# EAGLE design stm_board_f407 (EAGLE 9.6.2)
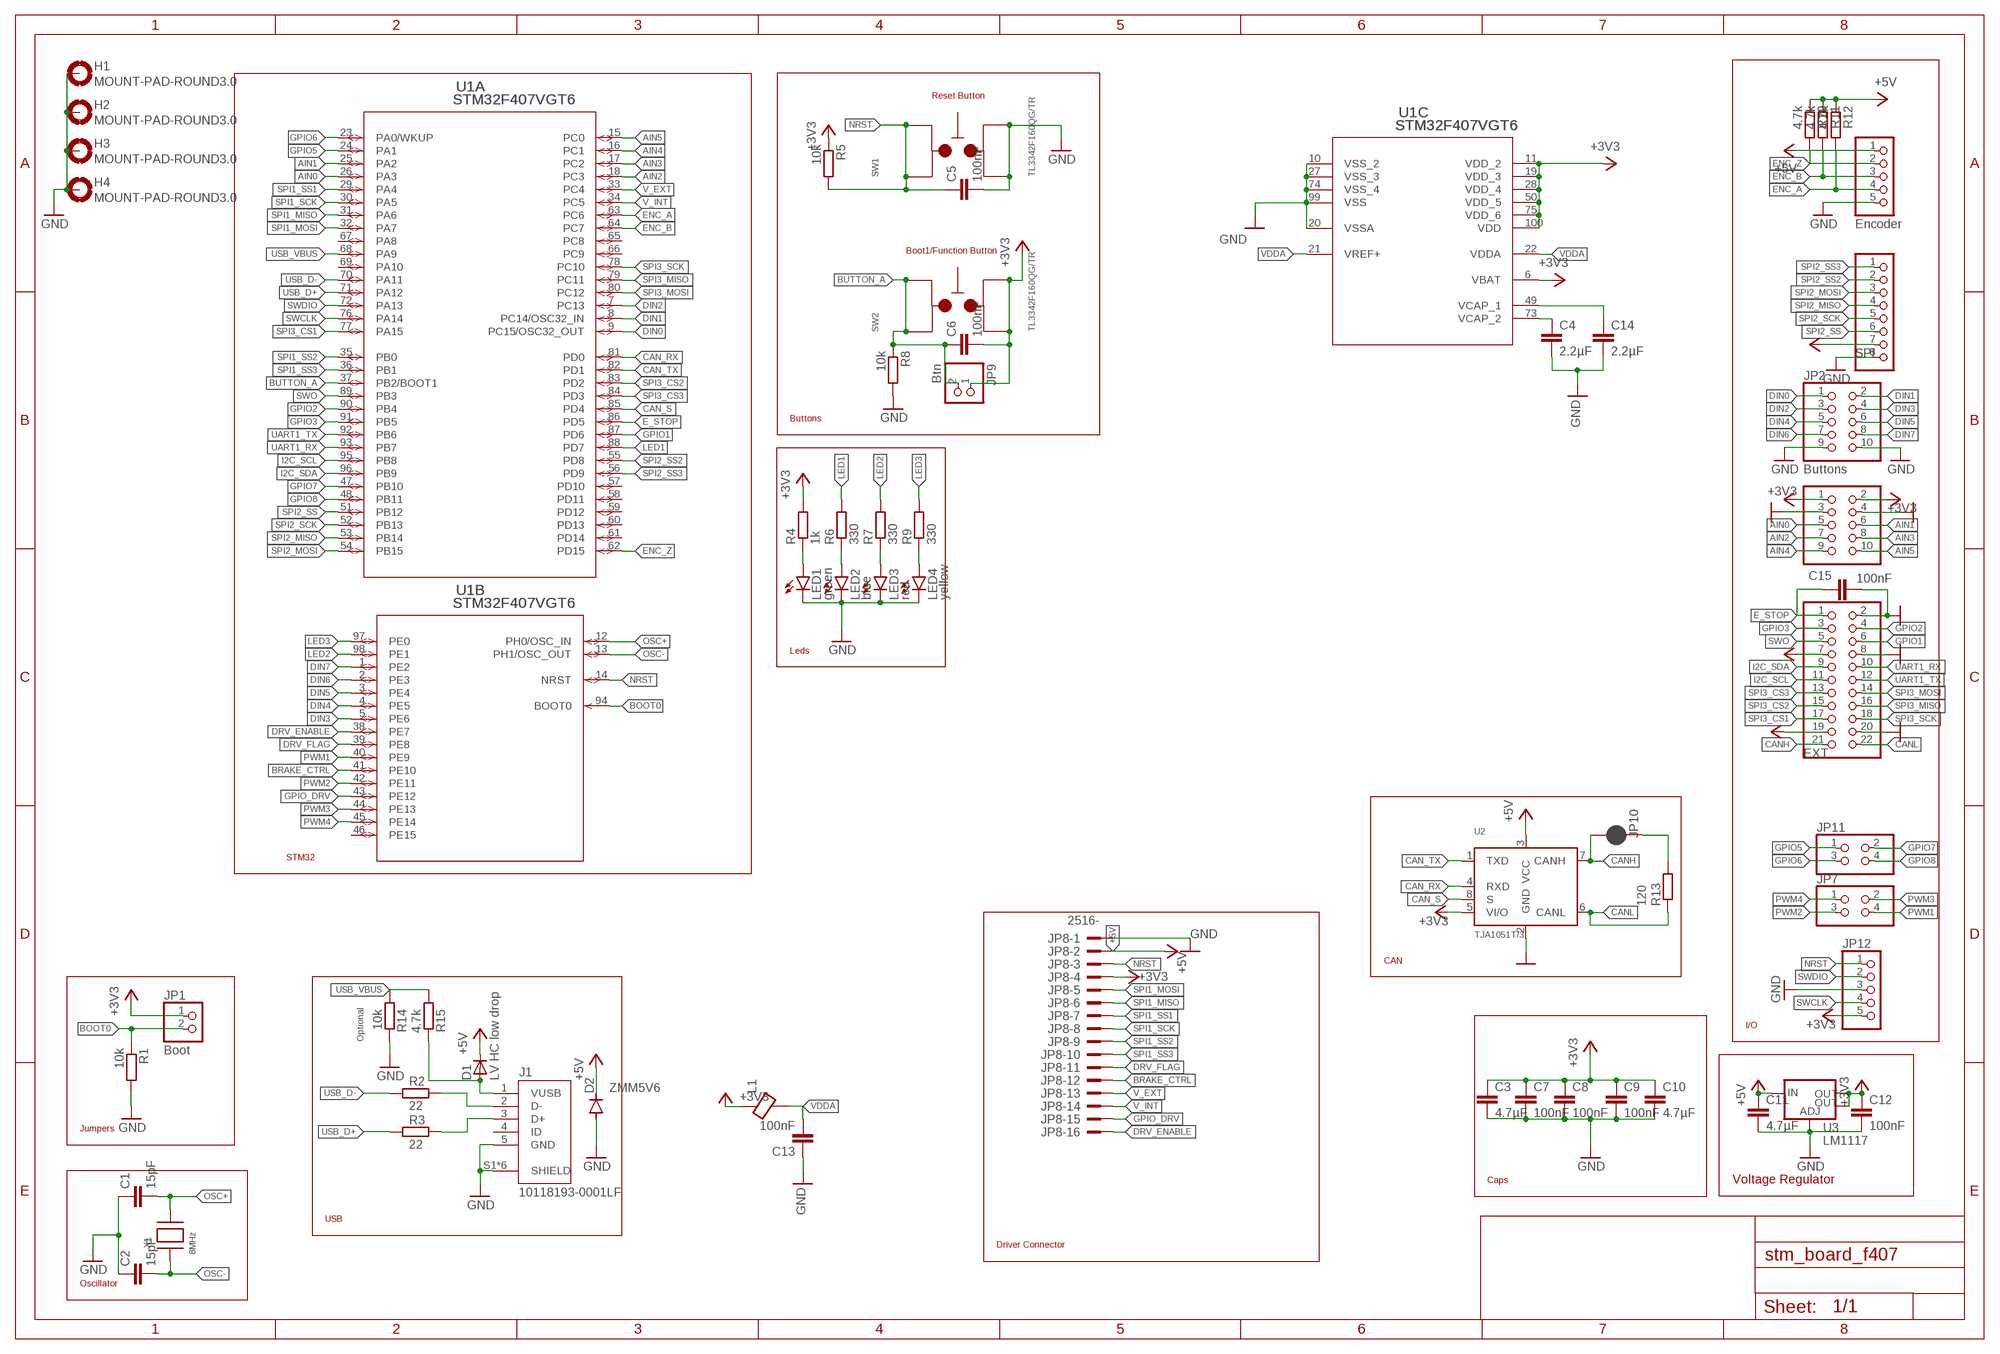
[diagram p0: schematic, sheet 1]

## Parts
C1  15pF  C-EUC0603  [C0603]
C2  15pF  C-EUC0603  [C0603]
C3  4.7µF  C-EUC0805  [C0805]
C4  2.2µF  C-EUC0603  [C0603]
C5  100nF  C-EUC0603  [C0603]
C6  100nF  C-EUC0603  [C0603]
C7  100nF  C-EUC0603  [C0603]
C8  100nF  C-EUC0603  [C0603]
C9  100nF  C-EUC0603  [C0603]
C10  4.7µF  C-EUC0805  [C0805]
C11  4.7µF  C-EUC0805  [C0805]
C12  100nF  C-EUC0603  [C0603]
C13  100nF  C-EUC0603  [C0603]
C14  2.2µF  C-EUC0603  [C0603]
C15  100nF  C-EUC0603  [C0603]
D1  LV HC low drop  DIODESMA  [SMADIODE]
D2  ZMM5V6  DIODE-MINIMELF  [MINIMELF]
H1  MOUNT-PAD-ROUND3.0  [3,0-PAD]
H2  MOUNT-PAD-ROUND3.0  [3,0-PAD]
H3  MOUNT-PAD-ROUND3.0  [3,0-PAD]
H4  MOUNT-PAD-ROUND3.0  [3,0-PAD]
J1  10118193-0001LF  [FCI_10118193-0001LF]
JP1  Boot  PINHD-1X2  [1X02]
JP2  Buttons  PINHD-2X5  [2X05]
JP3  Analog  PINHD-2X5  [2X05]
JP4  EXT  PINHD-2X11  [2X11]
JP5  Encoder  PINHD-1X5  [1X05]
JP6  SPI  PINHD-1X8  [1X08]
JP7  PINHD-2X2  [2X02]
JP8  2516-  [PAK100/2500-16]
JP9  Btn  PINHD-1X2  [1X02]
JP10  JUMPER-SMT_2_NC_PASTE_NO-SILK  [SMT-JUMPER_2_NC_PASTE_NO-SILK]
JP11  PINHD-2X2  [2X02]
JP12  PINHD-1X5  [1X05]
L1  GZ2012D601TF  BLM21PG331SN1D  [BLM21PG331SN1D]
LED1  green  LEDSML0805  [SML0805]
LED2  blue  LEDSML0805  [SML0805]
LED3  red  LEDSML0805  [SML0805]
LED4  yellow  LEDSML0805  [SML0805]
R1  10k  R-EU_R0603  [R0603]
R2  22  R-EU_R0603  [R0603]
R3  22  R-EU_R0603  [R0603]
R4  1k  R-EU_R0603  [R0603]
R5  10k  R-EU_R0603  [R0603]
R6  330  R-EU_R0603  [R0603]
R7  330  R-EU_R0603  [R0603]
R8  10k  R-EU_R0603  [R0603]
R9  330  R-EU_R0603  [R0603]
R10  4.7k  R-EU_R0603  [R0603]
R11  4.7k  R-EU_R0603  [R0603]
R12  4.7k  R-EU_R0603  [R0603]
R13  120  R-EU_R0603  [R0603]
R14  10k  R-EU_R0603  [R0603]
R15  4.7k  R-EU_R0603  [R0603]
SW1  TL3342F160QG/TR  [TL3342F160QG/TR]
SW2  TL3342F160QG/TR  [TL3342F160QG/TR]
U1  STM32F407VGT6  [LQFP100-14X14MM]
U2  TJA1051T/3  [SOT96-1]
U3  LM1117  V_REG_LM1117SOT223  [SOT223]
X1  8MHz  XTALNX5032  [NX5032]

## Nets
+3V3: C3.1 C6.2 C7.1 C8.1 C9.1 C10.1 C12.1 JP1.1 JP3.1 JP3.2 JP4.7 JP6.7 JP8.4 JP9.1 JP12.5 L1.1 R4.2 R5.1 SW2.1 SW2.2 U1.6(C:VBAT) U1.11(C:VDD_2) U1.19(C:VDD_3) U1.28(C:VDD_4) U1.50(C:VDD_5) U1.75(C:VDD_6) U1.100(C:VDD) U2.5(VI/O) U3.2(OUT) U3.4(OUT)
+5V: C11.1 D1.C D2.C JP4.19 JP5.1 JP8.2 R10.1 R11.1 R12.1 U2.3(VCC) U3.3(IN)
AIN0: JP3.5 U1.26(A:PA3)
AIN1: JP3.6 U1.25(A:PA2)
AIN2: JP3.7 U1.18(A:PC3)
AIN3: JP3.8 U1.17(A:PC2)
AIN4: JP3.9 U1.16(A:PC1)
AIN5: JP3.10 U1.15(A:PC0)
BOOT0: JP1.2 R1.1 U1.94(B:BOOT0)
BRAKE_CTRL: JP8.12 U1.41(B:PE10)
BUTTON_A: C6.1 JP9.2 R8.1 SW2.3 SW2.4 U1.37(A:PB2/BOOT1)
CAN_RX: U1.81(A:PD0) U2.4(RXD)
CAN_S: U1.85(A:PD4) U2.8(S)
CAN_TX: U1.82(A:PD1) U2.1(TXD)
CANH: JP4.21 JP10.2 U2.7(CANH)
CANL: JP4.22 R13.1 U2.6(CANL)
DIN0: JP2.1 U1.9(A:PC15/OSC32_OUT)
DIN1: JP2.2 U1.8(A:PC14/OSC32_IN)
DIN2: JP2.3 U1.7(A:PC13)
DIN3: JP2.4 U1.5(B:PE6)
DIN4: JP2.5 U1.4(B:PE5)
DIN5: JP2.6 U1.3(B:PE4)
DIN6: JP2.7 U1.2(B:PE3)
DIN7: JP2.8 U1.1(B:PE2)
DRV_ENABLE: JP8.16 U1.38(B:PE7)
DRV_FLAG: JP8.11 U1.39(B:PE8)
E_STOP: C15.1 JP4.1 U1.86(A:PD5)
ENC_A: JP5.4 R12.2 U1.63(A:PC6)
ENC_B: JP5.3 R11.2 U1.64(A:PC7)
ENC_Z: JP5.2 R10.2 U1.62(A:PD15)
GND: C1.1 C2.1 C3.2 C4.2 C5.2 C7.2 C8.2 C9.2 C10.2 C11.2 C12.2 C13.1 C14.2 C15.2 D2.A H1.B3,0(MOUNT) H2.B3,0(MOUNT) H3.B3,0(MOUNT) H4.B3,0(MOUNT) J1.5(GND) J1.S1(SHIELD) J1.S2(SHIELD) J1.S3(SHIELD) J1.S4(SHIELD) J1.S5(SHIELD) J1.S6(SHIELD) JP2.9 JP2.10 JP3.3 JP3.4 JP4.2 JP4.8 JP4.20 JP5.5 JP6.8 JP8.1 JP12.3 LED1.C LED2.C LED3.C LED4.C R1.2 R8.2 R14.2 SW1.1 SW1.2 U1.10(C:VSS_2) U1.20(C:VSSA) U1.27(C:VSS_3) U1.74(C:VSS_4) U1.99(C:VSS) U2.2(GND) U3.1(ADJ)
GPIO1: JP4.6 U1.87(A:PD6)
GPIO2: JP4.4 U1.90(A:PB4)
GPIO3: JP4.3 U1.91(A:PB5)
GPIO5: JP11.1 U1.24(A:PA1)
GPIO6: JP11.3 U1.23(A:PA0/WKUP)
GPIO7: JP11.2 U1.47(A:PB10)
GPIO8: JP11.4 U1.48(A:PB11)
GPIO_DRV: JP8.15 U1.43(B:PE12)
I2C_SCL: JP4.11 U1.95(A:PB8)
I2C_SDA: JP4.9 U1.96(A:PB9)
LED1: R6.2 U1.88(A:PD7)
LED2: R7.2 U1.98(B:PE1)
LED3: R9.2 U1.97(B:PE0)
N$1: D1.A J1.1(VUSB) R15.2
N$2: LED4.A R9.1
N$3: JP10.1 R13.2
N$4: C14.1 U1.49(C:VCAP_1)
N$5: J1.2(D-) R2.2
N$6: J1.3(D+) R3.2
N$7: C4.1 U1.73(C:VCAP_2)
N$11: LED1.A R4.1
N$12: LED2.A R6.1
N$13: LED3.A R7.1
NRST: C5.1 JP8.3 JP12.1 R5.2 SW1.3 SW1.4 U1.14(B:NRST)
OSC+: C1.2 U1.12(B:PH0/OSC_IN) X1.P$2
OSC-: C2.2 U1.13(B:PH1/OSC_OUT) X1.P$1
PWM1: JP7.4 U1.40(B:PE9)
PWM2: JP7.3 U1.42(B:PE11)
PWM3: JP7.2 U1.44(B:PE13)
PWM4: JP7.1 U1.45(B:PE14)
SPI1_MISO: JP8.6 U1.31(A:PA6)
SPI1_MOSI: JP8.5 U1.32(A:PA7)
SPI1_SCK: JP8.8 U1.30(A:PA5)
SPI1_SS1: JP8.7 U1.29(A:PA4)
SPI1_SS2: JP8.9 U1.35(A:PB0)
SPI1_SS3: JP8.10 U1.36(A:PB1)
SPI2_MISO: JP6.4 U1.53(A:PB14)
SPI2_MOSI: JP6.3 U1.54(A:PB15)
SPI2_SCK: JP6.5 U1.52(A:PB13)
SPI2_SS: JP6.6 U1.51(A:PB12)
SPI2_SS2: JP6.2 U1.55(A:PD8)
SPI2_SS3: JP6.1 U1.56(A:PD9)
SPI3_CS1: JP4.17 U1.77(A:PA15)
SPI3_CS2: JP4.15 U1.83(A:PD2)
SPI3_CS3: JP4.13 U1.84(A:PD3)
SPI3_MISO: JP4.16 U1.79(A:PC11)
SPI3_MOSI: JP4.14 U1.80(A:PC12)
SPI3_SCK: JP4.18 U1.78(A:PC10)
SWCLK: JP12.4 U1.76(A:PA14)
SWDIO: JP12.2 U1.72(A:PA13)
SWO: JP4.5 U1.89(A:PB3)
UART1_RX: JP4.10 U1.93(A:PB7)
UART1_TX: JP4.12 U1.92(A:PB6)
USB_D+: R3.1 U1.71(A:PA12)
USB_D-: R2.1 U1.70(A:PA11)
USB_VBUS: R14.1 R15.1 U1.68(A:PA9)
V_EXT: JP8.13 U1.33(A:PC4)
V_INT: JP8.14 U1.34(A:PC5)
VDDA: C13.2 L1.2 U1.21(C:VREF+) U1.22(C:VDDA)
Unconnected: J1.4(ID) U1.46(B:PE15) U1.57(A:PD10) U1.58(A:PD11) U1.59(A:PD12) U1.60(A:PD13) U1.61(A:PD14) U1.65(A:PC8) U1.66(A:PC9) U1.67(A:PA8) U1.69(A:PA10)

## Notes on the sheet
- Reset Button
- Boot1/Function Button
- Buttons
- Leds
- STM32
- CAN
- I/O
- Optional
- Jumpers
- Caps | Voltage Regulator
- USB
- Driver Connector
- Oscillator

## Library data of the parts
C1-C15 = resistor:C-EU: CAPACITOR, European symbol
D1 = adafruit:DIODE: Diode
D2 = diode:DIODE-: DIODE
H1-H4 = holes:MOUNT-PAD-ROUND: MOUNTING PAD, round
J1 = con_ampusb_10118193-0001LF:10118193-0001LF: Micro USB B Type Receptacle; AVAILABILITY: Unavailable; DESCRIPTION: Single Port 5 Contact Shielded SMT MICRO USB B-Type Receptacle; MF: Amphenol ICC; MP: 10118193-0001LF; PACKAGE: None; PRICE: None
JP1 JP9 = pinhead:PINHD-1X2: PIN HEADER
JP2 JP3 = pinhead:PINHD-2X5: PIN HEADER
JP4 = pinhead:PINHD-2X11: PIN HEADER
JP5 JP12 = pinhead:PINHD-1X5: PIN HEADER
JP6 = pinhead:PINHD-1X8: PIN HEADER
JP7 JP11 = pinhead:PINHD-2X2: PIN HEADER
JP8 = con-3m:2516-: 3M (TM) Pak 100 4-Wall Header Source: 3M; OC_FARNELL: unknown; OC_NEWARK: unknown
JP10 = SparkFun-Jumpers:JUMPER-SMT_2_NC_PASTE: Normally closed solder jumper
L1 = Thermistor_Inductors:BLM21PG331SN1D: FERRITE BEAD 330 OHM 0805 1LN; CREATED_BY: PCBLayout.com; DIGIKEY_PART_NUMBER: 490-5988-2-ND; MANUFACTURER: Murata Electronics North America; MPN: BLM21PG331SN1D; PACKAGE: 0805
LED1-LED4 = led:LED: LED
R1-R15 = resistor:R-EU_: RESISTOR, European symbol
SW1 SW2 = Switch:TL3342F160QG/TR: SWITCH TACTILE SPST-NO 0.05A 12V Manufacturer's datasheet; CREATED_BY: PCBLayout.com; DIGI_KEY_PART_NUMBER: EG2531CT-ND; MANUFACTURER: E-Switch; MPN: TL3342F160QG/TR; PACKAGE: SPST_NO
U1 = STM32:STM32F407VGT6; BUILT_BY: EMA_UL_Team; COPYRIGHT: Copyright (C) 2018 Accelerated Designs. All rights reserved; MANUFACTURER_PART_NUMBER: STM32F407VGT6; SOURCELIBRARY: Updates_to_database_2020-10-19; VENDOR: STMicroelectronics
U2 = TJA1051T_3:TJA1051T/3: High-speed CAN transceiver The TJA1051 is a high-speed CAN transceiver that provides an interface between a Controller Area Network (CAN) protocol controller and the physical two-wire CAN bus. The transceiver is designed for high-speed (up to 1 Mbit/s) CAN applications in the automotive industry,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; AVAILABILITY: Bad; DESCRIPTION: 1/1 Transceiver Half CANbus 8-SO; MF: NXP Semiconductors; MP: TJA1051T/3; PACKAGE: SOIC-8 NXP Semiconductors; PRICE: None
U3 = SparkFun-IC-Power:V_REG_LM1117: Voltage Regulator LM1117 Standard adjustable voltage regulator but in SMD form. Spark Fun Electronics SKU : COM-00595; PROD_ID: VREG-08170
X1 = adafruit:XTAL: Low cost SMT crystals, no capacitors included

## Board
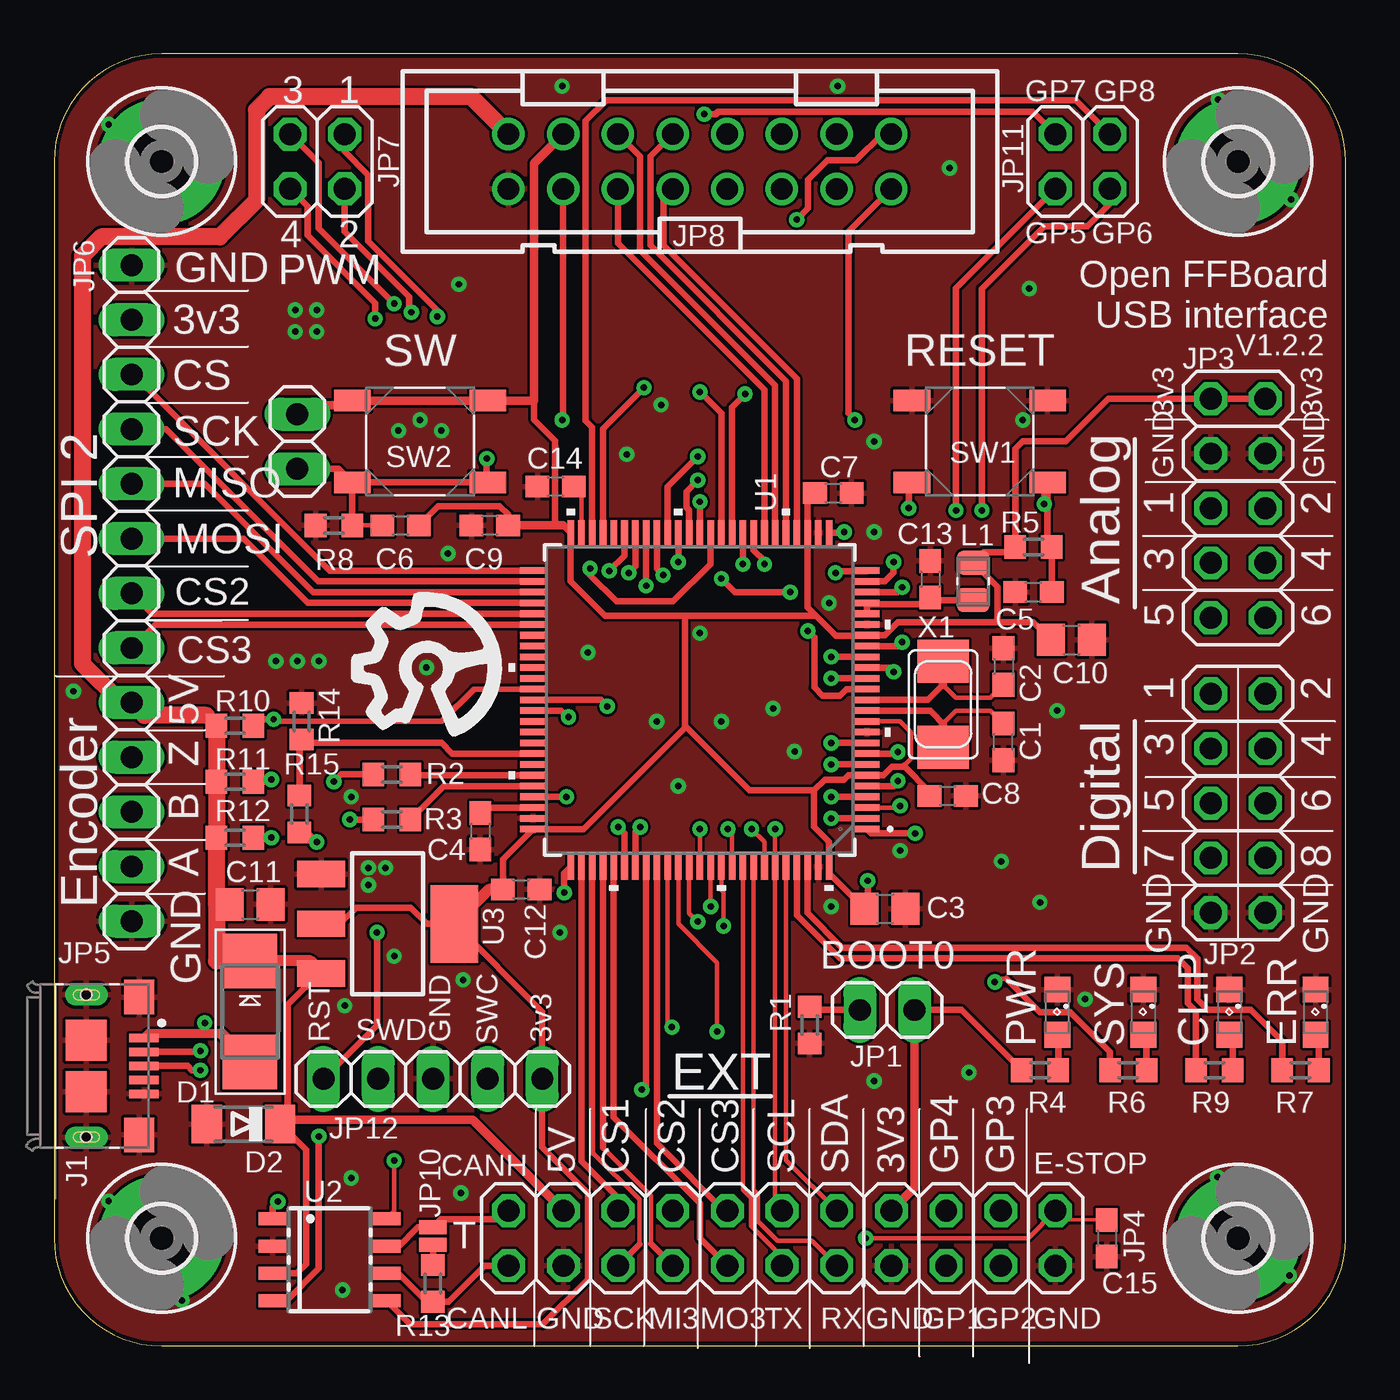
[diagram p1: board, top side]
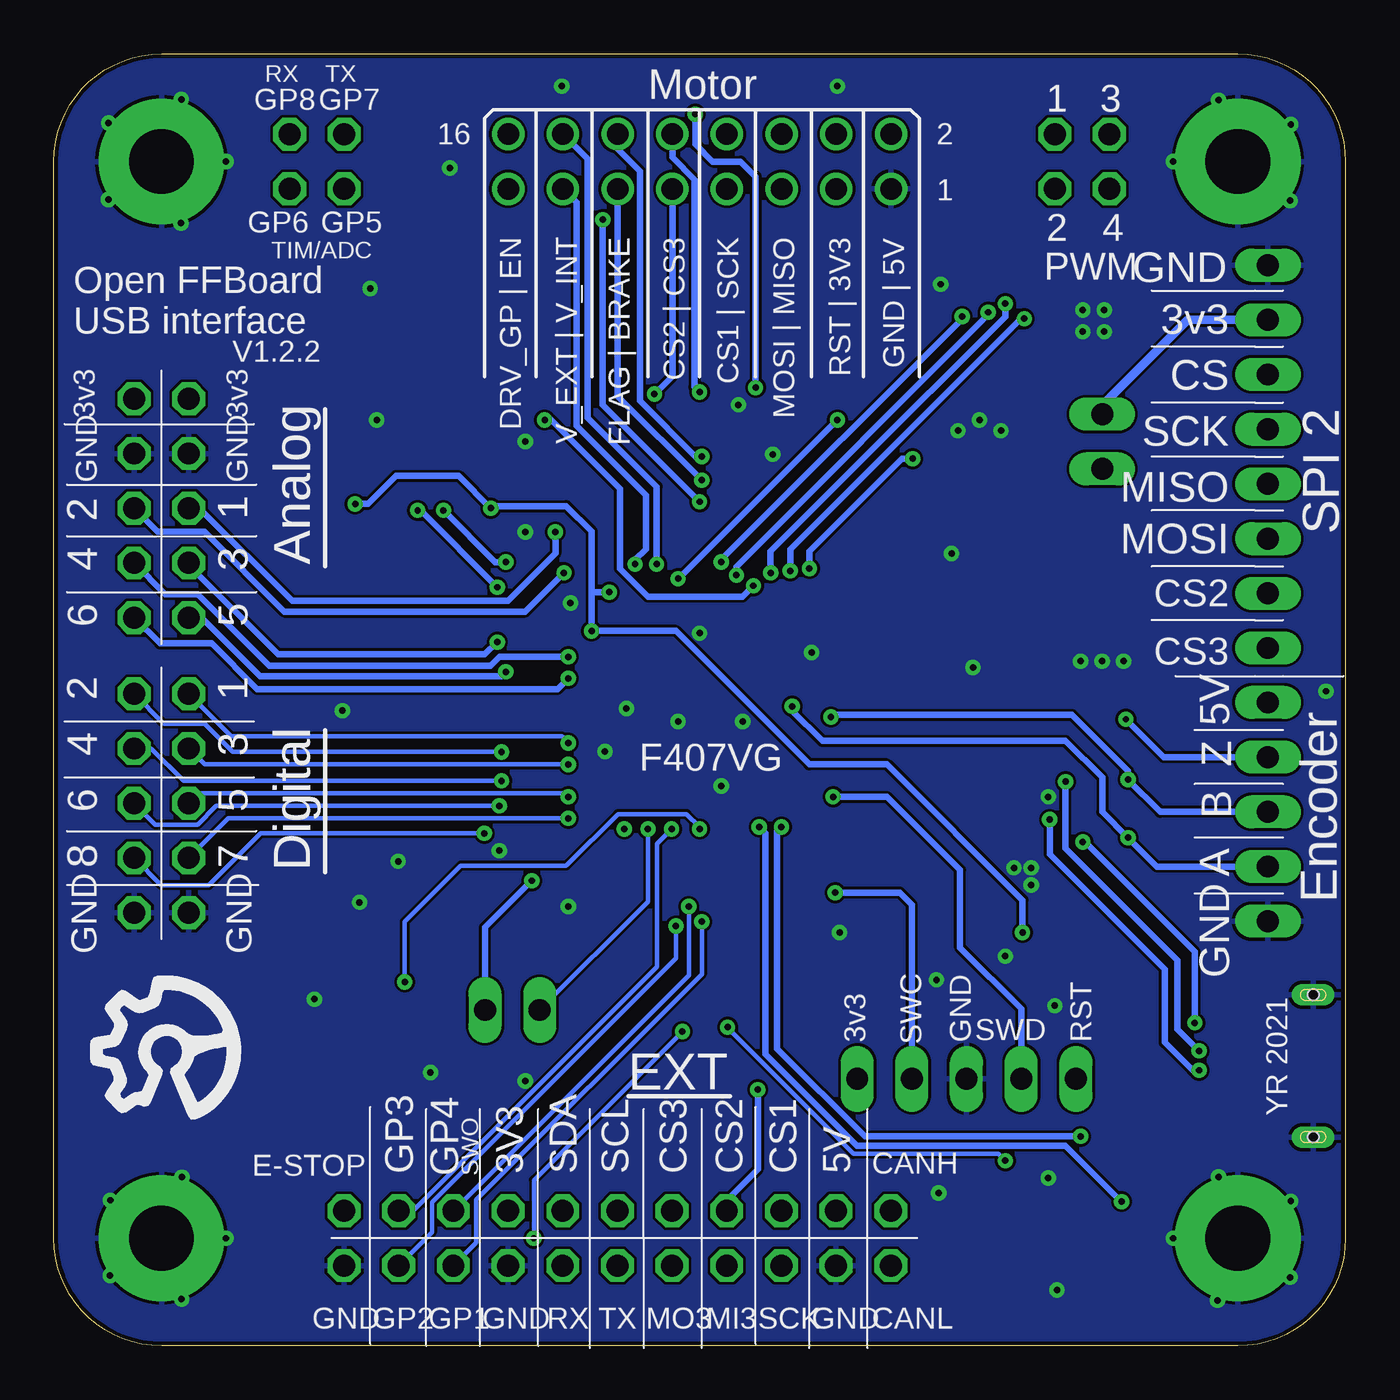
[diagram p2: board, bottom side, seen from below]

Size 60 x 60 mm. Coordinates in mm from the lower left corner, seen from the top.
Outline: 5,0 55,0 arc90 60,5 60,55 arc90 55,60 5,60 arc90 0,55 0,5 arc90 5,0
Copper layers (1*16): Top 0.035mm / dielectric 1.5mm / Bottom 0.035mm
Design rules "jlcpcb *": minimum track width 5mil, minimum drill 0.3mm, track to track 5mil, track to pad 5mil, pad to pad 5mil, via to via 5mil, smd to smd 5mil, copper to edge 0.2mm, drill to drill 8mil, minimum pad ring 10mil, minimum via ring 8mil, stop-mask expansion 2mil, vias tented up to drill 0.4mm, thermal gap 6mil

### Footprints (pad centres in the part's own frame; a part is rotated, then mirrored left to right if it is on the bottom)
C0603 = smd 1.1 x 1: 1 -0.85,0; 2 0.85,0
C0805 = smd 1.3 x 1.5: 1 -0.95,0; 2 0.95,0
SMADIODE = smd 2.54 x 2.54: A 2.349,0; C -2.349,0
MINIMELF = smd 1.4 x 1.8: A 1.7,0; C -1.7,0
3,0-PAD = drill 3 pad 5.842: B3,0 0,0
FCI_10118193-0001LF = smd 0.4 x 1.35: 1 -1.3,2.675; 2 -0.65,2.675; 3 0,2.675; 4 0.65,2.675; 5 1.3,2.675 | smd 1.6 x 1.4: S1 -3.2,2.45; S2 3.2,2.45 | smd 1.9 x 1.9: S3 1.2,0; S4 -1.2,0 | drill 0.5 pad 0.9 long: S5 -3.3,0; S6 3.3,0 | hole 0.5: -3.3,0; 3.3,0
1X02 = drill 1.016 long: 1 -1.27,0; 2 1.27,0
2X05 = drill 1.016 octagon: 1 -5.08,-1.27; 2 -5.08,1.27; 3 -2.54,-1.27; 4 -2.54,1.27; 5 0,-1.27; 6 0,1.27; 7 2.54,-1.27; 8 2.54,1.27; 9 5.08,-1.27; 10 5.08,1.27
2X11 = drill 1.016 octagon: 1 -12.7,-1.27; 2 -12.7,1.27; 3 -10.16,-1.27; 4 -10.16,1.27; 5 -7.62,-1.27; 6 -7.62,1.27; 7 -5.08,-1.27; 8 -5.08,1.27; 9 -2.54,-1.27; 10 -2.54,1.27; 11 0,-1.27; 12 0,1.27; 13 2.54,-1.27; 14 2.54,1.27; 15 5.08,-1.27; 16 5.08,1.27; 17 7.62,-1.27; 18 7.62,1.27; 19 10.16,-1.27; 20 10.16,1.27; 21 12.7,-1.27; 22 12.7,1.27
1X05 = drill 1.016 long: 1 -5.08,0; 2 -2.54,0; 3 0,0; 4 2.54,0; 5 5.08,0
1X08 = drill 1.016 long: 1 -8.89,0; 2 -6.35,0; 3 -3.81,0; 4 -1.27,0; 5 1.27,0; 6 3.81,0; 7 6.35,0; 8 8.89,0
2X02 = drill 1.016 octagon: 1 -1.27,-1.27; 2 -1.27,1.27; 3 1.27,-1.27; 4 1.27,1.27
PAK100/2500-16 = drill 1 pad 1.422: 1 -8.89,-1.27; 2 -8.89,1.27; 3 -6.35,-1.27; 4 -6.35,1.27; 5 -3.81,-1.27; 6 -3.81,1.27; 7 -1.27,-1.27; 8 -1.27,1.27; 9 1.27,-1.27; 10 1.27,1.27; 11 3.81,-1.27; 12 3.81,1.27; 13 6.35,-1.27; 14 6.35,1.27; 15 8.89,-1.27; 16 8.89,1.27
SMT-JUMPER_2_NC_PASTE_NO-SILK = smd 0.635 x 1.27: 1 -0.406,0; 2 0.406,0
BLM21PG331SN1D = smd 1.09 x 1.47: 1 -0.865,0; 2 0.865,0
SML0805 = smd 1.2 x 1.2: A 1.05,0; C -1.05,0
R0603 = smd 1 x 1.1: 1 -0.85,0; 2 0.85,0
TL3342F160QG/TR = smd 1.7 x 1: 1 -3.15,-1.9; 2 3.15,-1.9; 3 -3.15,1.9; 4 3.15,1.9
LQFP100-14X14MM = smd 0.305 x 1.194: 1 -6,-7.75; 2 -5.5,-7.75; 3 -5,-7.75; 4 -4.5,-7.75; 5 -4,-7.75; 6 -3.5,-7.75; 7 -3,-7.75; 8 -2.5,-7.75; 9 -2,-7.75; 10 -1.5,-7.75; 11 -1,-7.75; 12 -0.5,-7.75; 13 0,-7.75; 14 0.5,-7.75; 15 1,-7.75; 16 1.5,-7.75; 17 2,-7.75; 18 2.5,-7.75; 19 3,-7.75; 20 3.5,-7.75; 21 4,-7.75; 22 4.5,-7.75; 23 5,-7.75; 24 5.5,-7.75; 25 6,-7.75; 51 6,7.75; 52 5.5,7.75; 53 5,7.75; 54 4.5,7.75; 55 4,7.75; 56 3.5,7.75; 57 3,7.75; 58 2.5,7.75; 59 2,7.75; 60 1.5,7.75; 61 1,7.75; 62 0.5,7.75; 63 0,7.75; 64 -0.5,7.75; 65 -1,7.75; 66 -1.5,7.75; 67 -2,7.75; 68 -2.5,7.75; 69 -3,7.75; 70 -3.5,7.75; 71 -4,7.75; 72 -4.5,7.75; 73 -5,7.75; 74 -5.5,7.75; 75 -6,7.75 | smd 1.194 x 0.305: 26 7.75,-6; 27 7.75,-5.5; 28 7.75,-5; 29 7.75,-4.5; 30 7.75,-4; 31 7.75,-3.5; 32 7.75,-3; 33 7.75,-2.5; 34 7.75,-2; 35 7.75,-1.5; 36 7.75,-1; 37 7.75,-0.5; 38 7.75,0; 39 7.75,0.5; 40 7.75,1; 41 7.75,1.5; 42 7.75,2; 43 7.75,2.5; 44 7.75,3; 45 7.75,3.5; 46 7.75,4; 47 7.75,4.5; 48 7.75,5; 49 7.75,5.5; 50 7.75,6; 76 -7.75,6; 77 -7.75,5.5; 78 -7.75,5; 79 -7.75,4.5; 80 -7.75,4; 81 -7.75,3.5; 82 -7.75,3; 83 -7.75,2.5; 84 -7.75,2; 85 -7.75,1.5; 86 -7.75,1; 87 -7.75,0.5; 88 -7.75,0; 89 -7.75,-0.5; 90 -7.75,-1; 91 -7.75,-1.5; 92 -7.75,-2; 93 -7.75,-2.5; 94 -7.75,-3; 95 -7.75,-3.5; 96 -7.75,-4; 97 -7.75,-4.5; 98 -7.75,-5; 99 -7.75,-5.5; 100 -7.75,-6
SOT96-1 = smd 0.6 x 1.3: 1 -1.905,-2.65; 2 -0.635,-2.65; 3 0.635,-2.65; 4 1.905,-2.65; 5 1.905,2.65; 6 0.635,2.65; 7 -0.635,2.65; 8 -1.905,2.65
SOT223 = smd 1.219 x 2.235: 1 -2.311,-3.099; 2 0,-3.099; 3 2.311,-3.099 | smd 3.6 x 2.2: 4 0,3.099
NX5032 = smd 2 x 2.4: P$1 2,0; P$2 -2,0

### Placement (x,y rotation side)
C1  44.1,28.05 90 top
C2  44.1,31.55 270 top
C3  38.6,20.3 0 top
C4  19.8,23.9 270 top
C5  45.5,35 180 top
C6  16.1,38.1 0 top
C7  36.2,39.6 0 top
C8  41.51,25.54 0 top
C9  20.24,38.1 180 top
C10  47.26,32.79 0 top
C11  9.1,20.5 0 top
C12  21.7,21.2 0 top
C13  40.7,35.6 270 top
C14  23.3,39.9 180 top
C15  48.9,5 270 top
D1  9.1,15.53 270 top
D2  8.8,10.3 180 top
H1  55,5 0 top
H2  5,5 0 top
H3  55,55 0 top
H4  5,55 0 top
J1  1.5,13 270 top
JP1  38.7,15.6 180 top
JP2  55,25.2 270 top
JP3  55,38.9 270 top
JP4  33.82,5 180 top
JP5  3.6,24.8 270 top
JP6  3.6,41.3 90 top
JP7  12.23,55 0 top
JP8  30,55 0 top
JP9  11.3,42 270 top
JP10  17.6,5.1 90 top
JP11  47.78,55 0 top
JP12  17.6,12.4 0 top
L1  42.7,35.5 270 top
LED1  46.6,15.5 270 top
LED2  50.6,15.5 270 top
LED3  58.6,15.5 270 top
LED4  54.6,15.5 270 top
R1  35.1,14.9 270 top
R2  15.69,26.54 180 top
R3  15.69,24.44 180 top
R4  45.8,12.8 180 top
R5  45.5,37.1 0 top
R6  49.9,12.8 180 top
R7  57.9,12.8 180 top
R8  13,38.1 180 top
R9  53.9,12.8 180 top
R10  8.4,28.8 0 top
R11  8.4,26.2 0 top
R12  8.4,23.6 0 top
R13  17.6,2.9 90 top
R14  11.5,29 90 top
R15  11.4,24.7 270 top
SW1  43,42 180 top
SW2  17,42 180 top
U1  30,30 90 top
U2  12.8,4 270 top
U3  15.5,19.6 270 top
X1  41.3,29.8 90 top

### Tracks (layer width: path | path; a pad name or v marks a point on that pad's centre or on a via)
+3V3  (via drill 0.3)
  Top 0.2: C7.1 35,39.25 | 37.73,32.98 U1.19 | U1.11 39.3,29 39.8,28.5 39.8,27.26 39.47,26.93 39.44,26.9 | C8.1 40.66,25.74
  Top 0.3: JP3.2 JP3.1 48.98,43.98 47,42 45,42 44.65,41.65 R5.1 44.65,36.86 43.2,36.86 L1.1 | U1.75 20.85,22.6 C12.1 | 23.65,38.1 U1.50 | 35,39.25 U1.28 35,34.3 35.4,33.9 | 35.4,33.9 36.32,32.98 37.73,32.98 | 35.3,25.8 35.8,26.3 36.7,26.3 36.9,26.5 U1.6 38.52,26.5 38.92,26.9 39.44,26.9 | 35.3,25.8 35.3,24.1 36,23.4 U1.100 36,21.95 C3.1 37.8,20.45 v37.8,21.6 | 40.66,25.74 39.47,26.93 | 24,36.72 U1.50 | U1.75 24.6,24 29.3,28.7 | 29.3,28.7 29.35,28.75 32.3,25.8 35.3,25.8 | U1.50 24,35.5 25.6,33.9 29.28,33.9 29.29,33.89 | 42.5,36.56 L1.1 | U1.19 38.6,33 39.2,33.6 43.7,33.6 | 43.7,33.6 43.82,33.72 43.82,35.24 L1.1 | 35.4,33.9 29.3,33.9 29.29,33.89 | 29.3,28.7 29.3,33.88 29.29,33.89 | C10.1 45.5,33.6 43.7,33.6 | R4.2 42.15,15.6 JP1.1 | 23.28,38.1 23.28,42.02 22.3,43 22.3,43.9 | U2.5 16.55,1 22.7,1 24.8,3.1 24.8,7.1 22.68,9.22 JP12.5 22.68,15.52 U3.4 17.33,19.6 16.57,20.35 14.03,20.35 13.27,19.6 U3.2 | C6.2 17.85,39 20.7,39 21.09,38.61 C9.1 | U1.75 22.3,23.95
  Top 0.4: JP8.4 22.3,54.92 22.3,43.9 SW2.1 SW2.2 13.62,43.67 11.7,43.67 JP9.1 | 22.3,38.1 C9.1 23.28,38.1 23.65,38.1 | JP4.7 39.97,7.34 JP1.1
  Top 0.5: C12.1 20.2,21.2 U3.4
  Bottom 0.3: JP1.1 39.97,19.43 v37.8,21.6
  Bottom 0.4: JP9.1 11.3,43.67 7.32,47.65 JP6.7
+5V
  Top 0.3: 12.4,17.39 10.85,15.83 10.85,11.1 10.5,10.75 10.5,10.5 D2.C 11.7,9.1 11.7,3.8 11.27,3.37 U2.3
  Top 0.4: JP4.19 19.43,10.5 10.5,10.5
  Top 0.5: R12.1 7.5,23.6 7.46,23.56 | 7.07,29.28 R10.1 | D1.C 11.91,17.88 12.4,17.39 U3.3 | C11.1 7.55,20.5
  Top 0.8: R10.1 R11.1 R12.1 7.55,20.5 7.55,17.88 D1.C | 7.07,29.28 4.2,29.28 JP5.1 3.12,29.88 1.31,31.69 1.31,50.61 2.2,51.5 7.7,51.5 9.4,53.2 9.4,57.4 10.01,58.01 19.37,58.01 JP8.2
AIN0  (via drill 0.3)
  Top 0.2: 36.65,37.75 v36.7,37.8
  Top 0.3: U1.26 36.65,37.75
  Bottom 0.3: v36.7,37.8 36.7,36.8 38.9,34.6 48.94,34.6 53.24,38.9 JP3.5
AIN1  (via drill 0.3)
  Top 0.2: 37.73,35.98 U1.25
  Top 0.3: 37.73,35.98 36.56,35.98 36.48,35.9 v36.3,35.9
  Bottom 0.3: JP3.6 55.17,37.8 53,37.8 49.3,34.1 38.1,34.1 v36.3,35.9
AIN2  (via drill 0.3)
  Top 0.3: U1.18 39.22,32.5 v39.4,32.68
  Bottom 0.2: 53.73,36.26 JP3.7
  Bottom 0.3: v39.4,32.68 39.42,32.68 39.99,32.11 49.58,32.11 53.73,36.26
AIN3  (via drill 0.3)
  Top 0.3: U1.17 v36.1,32
  Bottom 0.3: JP3.8 54.82,34.91 53.32,34.91 49.99,31.58 39.72,31.58 39.3,32 v36.1,32
AIN4  (via drill 0.3)
  Top 0.3: v39,31.3 38.8,31.5 U1.16
  Bottom 0.2: JP3.9 53.13,33.82
  Bottom 0.3: 53.13,33.82 50.41,31.1 39.2,31.1 v39,31.3
AIN5  (via drill 0.3)
  Top 0.3: U1.15 v36.1,31
  Bottom 0.3: v36.1,31 36.6,30.5 50.55,30.5 52.67,32.62 55.07,32.62 JP3.10
BOOT0  (via drill 0.3)
  Top 0.2: U1.94 33,23.4 v32.4,24
  Top 0.3: JP1.2 35.25,15.6 R1.1
  Bottom 0.2: v32.4,24 32.4,20.63 JP1.2
BRAKE_CTRL  (via drill 0.3)
  Top 0.3: U1.41 28.5,39.9 v29.9,41.3
  Bottom 0.3: v29.9,41.3 30.19,41.3 32.78,43.89 32.78,54.56 33.81,55.59 JP8.12
BUTTON_A  (via drill 0.3)
  Top 0.2: C6.1 R8.1
  Top 0.3: v24.9,36.1 24.9,35.79 26.12,34.57 28.76,34.57 30.5,36.31 U1.37 | v20.1,41.2 20.1,40.15 SW2.3 SW2.4 | JP9.2 13.22,40.73 SW2.4 | SW2.4 R8.1
  Bottom 0.3: v24.9,36.1 24.9,36.9 20.6,41.2 v20.1,41.2
CAN_RX  (via drill 0.3)
  Top 0.3: v26.2,24.1 26.5,23.8 U1.81 | U2.4 10.8,2.09 12.3,3.6 v12.3,9.73
  Bottom 0.3: v26.2,24.1 26.4,23.9 26.4,13.8 22.33,9.73 v12.3,9.73
CAN_S  (via drill 0.3)
  Top 0.2: U2.8 15.8,6.26 v15.8,8.6 | U1.85 28.5,15 v28.7,14.8
  Bottom 0.2: v15.8,8.6 16.12,8.92 22.86,8.92 28.7,14.77 v28.7,14.8
CAN_TX  (via drill 0.3)
  Top 0.3: U2.1 10.15,6.45 v10.4,6.7 | v27.23,24.1 27,23.87 U1.82
  Bottom 0.3: v10.4,6.7 13,9.3 22.7,9.3 26.93,13.53 26.93,23.8 v27.23,24.1
CANH
  Top 0.3: U2.7 16.02,4.63 16.89,5.51 JP10.2 17.96,5.87 20.71,5.87 JP4.21
CANL
  Top 0.3: U2.6 15.98,3.37 17.3,2.05 R13.1 18.33,2.05 20.01,3.73 JP4.22
DIN0  (via drill 0.3)
  Top 0.3: v36.1,28 U1.9
  Bottom 0.2: JP2.1 51.75,28.3 36.4,28.3 v36.1,28
DIN1  (via drill 0.3)
  Top 0.2: 39.12,27.5 v39.2,27.58
  Top 0.3: U1.8 39.12,27.5
  Bottom 0.2: v39.2,27.58 51.68,27.58 53,28.9 54.89,28.9 JP2.2
DIN2  (via drill 0.3)
  Top 0.3: v36.1,27 U1.7
  Bottom 0.2: JP2.3 52.99,27 v36.1,27
DIN3  (via drill 0.3)
  Top 0.2: 39.2,26.18 v39.2,26.24
  Top 0.3: 39.2,26.18 39.02,26 U1.5
  Bottom 0.2: v39.2,26.24 53.97,26.24 55.47,27.74 JP2.4
DIN4  (via drill 0.3)
  Top 0.3: v36.1,25.5 U1.4
  Bottom 0.2: v36.1,25.5 36.26,25.66 53.27,25.66 JP2.5
DIN5  (via drill 0.3)
  Top 0.2: U1.3 39.22,25 v39.3,25.08
  Bottom 0.2: v39.3,25.08 52.45,25.08 53.32,24.21 55.28,24.21 JP2.6
DIN6  (via drill 0.3)
  Top 0.3: v36.1,24.5 U1.2
  Bottom 0.2: JP2.7 51.89,24.5 v36.1,24.5
DIN7  (via drill 0.3)
  Top 0.3: v40,23.8 37.95,23.8 U1.1
  Bottom 0.2: v40,23.8 50.4,23.8 52.8,21.4 55.01,21.4 JP2.8
DRV_ENABLE  (via drill 0.3)
  Top 0.3: U1.38 v30,39.2 | JP8.16 38.47,56.27 37.26,55.06 35.92,55.06 35.02,54.16 35.02,52.82 v34.5,52.3
  Bottom 0.3: v30,39.2 34.5,43.7 v34.5,52.3
DRV_FLAG  (via drill 0.3)
  Top 0.3: U1.39 29.5,38.81 29.37,38.94 29.37,39.67 v29.9,40.2
  Bottom 0.3: v29.9,40.2 33.81,44.11 JP8.11
E_STOP  (via drill 0.3)
  Top 0.152: JP4.1 46.94,5.85 C15.1
  Top 0.2: U1.86 29,19.6 30.8,17.8 v30.8,14.6 | v37.7,5 45.25,5 JP4.1
  Bottom 0.2: v30.8,14.6 37.7,7.7 v37.7,5
ENC_A  (via drill 0.3)
  Top 0.3: U1.63 25.4,30 v25.7,29.7 | v10.1,23.6 R12.2
  Bottom 0.3: JP5.4 8.76,22.26 v10.1,23.6 11.3,24.8 11.3,26.4 13,28.1 24.3,28.1 25.7,29.5 v25.7,29.7
ENC_B  (via drill 0.3)
  Top 0.3: U1.64 23.55,29.5 23.85,29.2 v23.9,29.2 | v10.1,26.3 10,26.2 R11.2
  Bottom 0.3: v23.9,29.2 23.8,29.3 12.7,29.3 10.1,26.7 v10.1,26.3 8.6,24.8 JP5.3
ENC_Z  (via drill 0.3)
  Top 0.254: U1.62 19.5,30.5 18,29 10.3,29 v10.2,29.1
  Top 0.3: 9.45,29 R10.2 9.55,29.1 v10.2,29.1
  Bottom 0.3: JP5.2 8.44,27.34 v10.2,29.1
GND  (via drill 0.3)
  other vias: 45,43 17,43 19,17 15.4,22.2 18.8,49.3 23.6,58.5 36.4,58.5 36.1,20.4 14.6,22.2 28.2,43.7 26.6,41.4 13.8,25.5 52,5 54.05,7.84 57.38,6.76 57.39,3.27 54.06,2.18 52,55 54.08,57.88 57.45,56.79 57.46,53.24 54.09,52.14 8,55 2.57,53.18 2.54,56.72 5.89,57.85 8,5 5.94,2.12 2.57,3.18 2.54,6.72 5.89,7.85 39.3,23 36,34.5 28,29 31,29 29,26 47.9,16.1 24.8,32.2 33.4,29.6 12.2,47.1 11.3,31.8 13.4,2.6 42.5,12.7 45.8,20.6 46.6,29.5 38.1,37.8 38.1,42 41.6,54.7 45.3,49.1 18.3,36.8 17.3,31.5 10.3,31.8 12.3,31.8 23.5,19.2 38.1,12.3 13.8,7.8 0.9,30.4 34.4,27.6 30,33.1 12.2,48.1 11.2,48.1 11.2,47.1 16,42.5 18,42.5 44,22.5 18.9,7.1 14.6,21.4 15.8,18.1 13.5,15.8
  pour Top: -1,61 -1,-1 61,-1 61,61
  pour Bottom: -2,61 -2,-1 60,-1 60,61
GPIO1  (via drill 0.3)
  Top 0.2: U1.87 29.5,20.1 v29.9,19.7
  Bottom 0.2: v29.9,19.7 29.9,17.27 40.39,6.78 40.39,4.78 JP4.6
GPIO2  (via drill 0.3)
  Top 0.2: U1.90 31,21.15 31.1,21.05 v31.1,19.5
  Bottom 0.2: JP4.4 42.43,5.28 42.43,6.68 31.1,18.01 v31.1,19.5
GPIO3  (via drill 0.3)
  Top 0.2: U1.91 31.5,23.8 v31.3,24
  Bottom 0.2: v31.3,24 31.98,23.32 31.98,17.6 43.31,6.27 JP4.3
GPIO5  (via drill 0.3)
  Top 0.3: U1.24 38.6,35.5 39,35.9 v39,36.4 | JP11.1 41.9,49.12 v41.9,38.8
  Bottom 0.3: v41.9,38.8 39.5,36.4 v39,36.4
GPIO6  (via drill 0.3)
  Top 0.3: U1.23 39.17,35 v39.4,35.23 | v43.1,38.8 43.1,49.1 46,52 48,52 49.05,53.05 JP11.3
  Bottom 0.3: v39.4,35.23 42.97,38.8 v43.1,38.8
GPIO7  (via drill 0.3)
  Top 0.3: JP11.2 45.48,57.3 30.84,57.3 30.74,57.2 v30.2,57.2 | v27.4,44.5 25.5,42.6 U1.47
  Bottom 0.3: v30.2,57.2 30.2,55.8 29.4,55 28.1,55 27.4,54.3 v27.4,44.5
GPIO8
  Top 0.3: U1.48 25,42.65 24.7,42.95 24.7,56.9 25.66,57.85 47.47,57.85 JP11.4
GPIO_DRV  (via drill 0.3)
  Top 0.3: U1.43 v27.5,35.3 | v37.2,43 36.9,43.3 36.9,51.74 JP8.15
  Bottom 0.3: v27.5,35.3 28,34.8 32.4,34.8 33.7,36.1 33.7,39.8 36.9,43 v37.2,43
I2C_SCL  (via drill 0.3)
  Top 0.2: v33.5,24 U1.95 33.5,6.59 JP4.11
I2C_SDA
  Top 0.2: U1.96 34,8.63 JP4.9
LED1  (via drill 0.3)
  Top 0.2: U1.88 v30,24 | 44.25,17.05 43.85,17.05 v43.7,16.9
  Top 0.3: R6.2 49.05,13.65 47.2,15.5 45.8,15.5 44.25,17.05
  Bottom 0.2: v30,24 30,24.1 30.6,24.7 33.8,24.7 36.2,22.3 41.1,22.3 43.7,19.7 v43.7,16.9
LED2
  Top 0.3: R7.2 57.05,14.15 55.6,15.6 53.6,15.6 53.1,16.1 53.1,18 52.6,18.5 36.61,18.5 35,20.11 U1.98
LED3
  Top 0.3: U1.97 34.5,20.01 36.51,18 52.2,18 52.67,17.53 52.67,15.92 53.05,15.55 R9.2
N$1  (via drill 0.3)
  Top 0.3: 7,14.5 v7,15 | v12.2,23.4 11.75,23.85 R15.2
  Top 0.406: 7.78,14.5 7,14.5 4.38,14.5 J1.1
  Top 0.5: D1.A 7.78,14.5
  Bottom 0.3: v7,15 7,18.3 12.1,23.4 v12.2,23.4
N$2
  Top 0.2: LED4.A 54.75,14.45
  Top 0.3: R9.1 54.75,14.45
N$3
  Top 0.3: R13.2 JP10.1
N$4
  Top 0.2: U1.49 24.5,39.55 C14.1
N$5  (via drill 0.3)
  Top 0.3: v6.8,13.7 6.75,13.65 J1.2 | v13,26.2 13.34,26.54 R2.2
  Bottom 0.3: v6.8,13.7 7.8,14.7 7.8,17.9 13,23.1 v13,26.2
N$6  (via drill 0.3)
  Top 0.3: R3.2 v13.74,24.44 | v6.8,12.8 6.4,12.8 6.2,13 J1.3
  Bottom 0.3: v6.8,12.8 7.1,12.8 8.4,14.1 8.4,17.5 13.74,22.84 v13.74,24.44
N$7
  Top 0.2: 20.05,25 C4.1
  Top 0.3: U1.73 20.05,25
N$11
  Top 0.2: LED1.A 46.65,14.4
  Top 0.3: R4.1 46.65,14.4
N$12
  Top 0.2: LED2.A 50.75,14.3
  Top 0.3: R6.1 50.75,14.3
N$13
  Top 0.2: LED3.A 58.75,14.3
  Top 0.3: R7.1 58.75,14.3
NRST  (via drill 0.3)
  Top 0.2: 39.7,39.95 SW1.4 40.35,40.1
  Top 0.3: U1.14 36.8,30.5 36.5,30.2 35.7,30.2 35.32,30.58 35.32,32.9 v35.02,33.2 | v39.7,38.9 39.7,39.95 | C5.1 R5.2 46.15,37.3 SW1.3 46,39.95 v46,39.1 | JP8.3 23.65,43.05 v23.6,43 | v31,35.63 31.63,35 v34.2,35 | JP12.1 15,14.88 v15,19.2
  Bottom 0.3: 35.02,35 35.02,37.82 36.2,39 39.6,39 v39.7,38.9 41.2,40.4 44.1,40.4 45.4,39.1 v46,39.1 | 35.02,35 v35.02,33.2 31.1,33.2 24.9,27 21.3,27 15,20.7 v15,19.2 | v31,35.63 30.97,35.63 v23.6,43 | v34.2,35 35.02,35
OSC+
  Top 0.2: C1.2 43.5,29.5 41.9,29.5 41.3,28.9
  Top 0.3: 41.3,28.9 40.8,29.4 40.7,29.5 U1.12
  Top 0.4: X1.P$2 41.3,28.9
OSC-
  Top 0.2: C2.2 43.5,30.1 41.9,30.1 41.3,30.7
  Top 0.3: U1.13 40.6,30 41.3,30.7
  Top 0.4: X1.P$1 41.3,30.7
PWM1  (via drill 0.3)
  Top 0.3: JP7.4 13.5,55.47 14.6,54.37 14.6,51.3 17.8,48.1 v17.8,47.8 | v29,36.4 U1.40
  Bottom 0.3: v17.8,47.8 17.8,47.7 29,36.5 v29,36.4
PWM2  (via drill 0.3)
  Top 0.2: v16.6,48 16.5,48.1
  Top 0.3: U1.42 28,36.08 v28.29,35.79 | 16.5,48.1 16.5,48.73 13.5,51.73 JP7.3
  Bottom 0.2: 16.6,47.88 v16.6,48
  Bottom 0.3: v28.29,35.79 28.29,36.19 16.6,47.88
PWM3  (via drill 0.3)
  Top 0.3: JP7.2 12.3,54.93 12.3,51.9 v15.8,48.4 | U1.44 27,36.2 v26.7,35.9
  Bottom 0.3: v15.8,48.4 15.8,47.8 22.8,40.8 26.7,36.9 v26.7,35.9
PWM4  (via drill 0.3)
  Top 0.3: U1.45 26.5,36.7 v25.79,35.99 | v14.92,47.7 14.92,48.42 11.77,51.56 11.77,52.92 JP7.1
  Bottom 0.3: v25.79,35.99 25.79,36.99 15.08,47.7 v14.92,47.7
SPI1_MISO
  Top 0.3: U1.31 33.5,44.6 27.22,50.88 27.22,55.24 JP8.6
SPI1_MOSI
  Top 0.3: U1.32 33,44.4 26.19,51.21 JP8.5
SPI1_SCK
  Top 0.3: U1.30 34,44.8 27.7,51.1 27.7,55.24 JP8.8
SPI1_SS1
  Top 0.3: U1.29 34.5,44.9 28.3,51.1 28.3,53.3 JP8.7
SPI1_SS2  (via drill 0.3)
  Top 0.3: v32.1,44.2 31.5,43.6 U1.35
  Bottom 0.3: JP8.9 31.27,45.03 v32.1,44.2
SPI1_SS3  (via drill 0.3)
  Top 0.3: v30,44.3 v30.01,44.3 31,43.31 U1.36
  Bottom 0.3: JP8.10 31.27,55.19 30.24,54.16 30.24,44.54 v30,44.3
SPI2_MISO
  Top 0.3: JP6.4 7,40.03 12.03,35 U1.53
SPI2_MOSI
  Top 0.3: JP6.3 8.8,37.49 11.79,34.5 U1.54
SPI2_SCK
  Top 0.3: U1.52 12.27,35.5 5.2,42.57 JP6.5
SPI2_SS
  Top 0.3: JP6.6 3.7,45.11 12.81,36 U1.51
SPI2_SS2
  Top 0.3: U1.55 4.55,34 JP6.2
SPI2_SS3
  Top 0.3: U1.56 4.69,33.5 JP6.1
SPI3_CS1
  Top 0.3: JP4.17 26.2,6.87 24.5,8.57 U1.77
SPI3_CS2  (via drill 0.3)
  Top 0.3: U1.83 27.5,12.1 v27.3,11.9
  Bottom 0.3: v27.3,11.9 27.3,8.21 28.74,6.77 JP4.15
SPI3_CS3
  Top 0.3: U1.84 28,9.4 31.28,6.12 JP4.13
SPI3_MISO
  Top 0.2: 27.73,4.74 27.73,6.98 25.5,9.2
  Top 0.3: U1.79 25.5,9.2 | JP4.16 27.73,4.74
SPI3_MOSI
  Top 0.3: U1.80 26,10.63 30.02,6.62 30.02,4.99 JP4.14
SPI3_SCK
  Top 0.2: 25,9 27.2,6.8 27.2,4.73
  Top 0.3: U1.78 25,9 | 27.2,4.73 JP4.18
SWCLK  (via drill 0.3)
  Top 0.3: U1.76 23.7,21.95 v23.7,21.05
  Bottom 0.3: v23.7,21.05 20.7,21.05 20.14,20.48 JP12.4
SWDIO  (via drill 0.3)
  Top 0.3: U1.72 v23.8,25.5
  Bottom 0.3: v23.8,25.5 21.3,25.5 17.9,22.1 17.9,18.5 15.06,15.66 JP12.2
SWO  (via drill 0.3)
  Top 0.2: U1.89 v30.5,20.4
  Bottom 0.2: v30.5,20.4 30.5,17.21 JP4.5
UART1_RX
  Top 0.2: JP4.10 35.21,4.88 33.61,4.88 32.7,5.79 32.7,7.05 32.5,7.25 U1.93
UART1_TX
  Top 0.2: JP4.12 33.82,4.13 32.37,5.58 32.37,6.88 32,7.25 U1.92
USB_D+
  Top 0.3: R3.1 18.1,26 U1.71
USB_D-
  Top 0.2: 16.54,26.65 R2.1 16.58,26.5
  Top 0.3: U1.70 16.58,26.5
USB_VBUS
  Top 0.3: R15.1 11.4,28.05 R14.1 11.65,28 18,28 18.5,27.5 U1.68
V_EXT  (via drill 0.3)
  Top 0.3: v33,36.3 33,36.45 32.5,36.95 U1.33
  Bottom 0.3: JP8.13 35.73,53.11 35.73,42.74 32.5,39.51 32.5,37 33,36.5 v33,36.3
V_INT  (via drill 0.3)
  Top 0.3: U1.34 v32,36.3
  Bottom 0.3: v32,36.3 32,39.9 35.2,43.1 35.2,55.12 JP8.14
VDDA
  Top 0.2: U1.21 U1.22 | C13.2 40.4,34.45 | 37.8,34.45 37.75,34.4
  Top 0.3: 40.4,34.45 37.8,34.45 | U1.21 37.75,34.4 | C13.2 40.81,34.64 L1.2

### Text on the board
tPlace: 3 | 1 | GP7 | GP8 | 4 | 2 | GP5 | GP6 | Open FFBoard / USB interface | GND | PWM | 3v3 | V1.2.2 | SW | RESET | CS | 3v3 | 3v3 | SPI 2 | SCK | GND | GND | MISO | 1 | 2 | Analog | MOSI | 3 | 4 | CS2 | 5 | 6 | CS3 | 1 | 2 | Encoder | 5V | Z | 3 | 4 | Digital | 5 | 6 | B | A | 7 | 8 | BOOT0 | GND | GND | GND | RST | SWD | GND | SWC | 3v3 | PWR | SYS | CLIP | ERR | EXT | CANH | 5V | CS1 | CS2 | CS3 | SCL | SDA | 3V3 | GP4 | GP3 | E-STOP | T | CANL | GND | SCK | MI3 | MO3 | TX | RX | GND | GP1 | GP2 | GND
bPlace: TX | RX | Motor | 3 | 1 | GP7 | GP8 | 2 | 16 | 1 | RST | 3V3 | MOSI | MISO | CS1 | SCK | CS2 | CS3 | FLAG | BRAKE | V_EXT | V_INT | DRV_GP | EN | GP5 | GP6 | GND | 4 | 2 | GND | 5V | PWM | TIM/ADC | 3v3 | V1.2.2 | Open FFBoard / USB interface | CS | SCK | 3v3 | 3v3 | MISO | Analog | GND | GND | SPI 2 | MOSI | 1 | 2 | CS2 | 3 | 4 | CS3 | 5 | 6 | 1 | 2 | 5V | Z | F407VG | 3 | 4 | Digital | 5 | 6 | B | A | 7 | 8 | Encoder | GND | GND | GND | SWD | RST | GND | SWC | 3v3 | EXT | YR 2021 | E-STOP | CANH | 5V | CS1 | CS2 | CS3 | SCL | SDA | 3V3 | SWO | GP4 | GP3 | CANL | GND | SCK | MI3 | MO3 | TX | RX | GND | GP1 | GP2 | GND

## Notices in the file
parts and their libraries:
SparkFun-IC-Power: Licensing: Creative Commons ShareAlike 4.0 International - https://creativecommons.org/licenses/by-sa/4.0
